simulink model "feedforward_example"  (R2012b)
settings: Solver=ode45  StartTime=0.0  StopTime=10.0  RelTol=1e-3
libraries: simulink x2

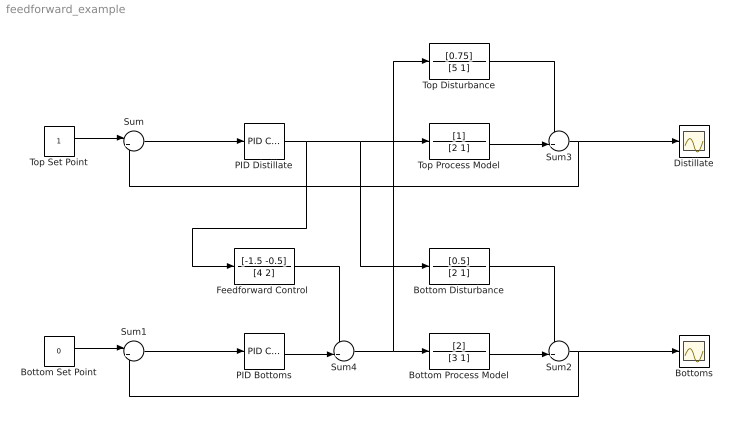
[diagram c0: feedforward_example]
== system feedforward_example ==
  Bottom Disturbance : TransferFcn  Numerator=[0.5]  Denominator=[2 1]
  Bottom Process Model : TransferFcn  Numerator=[2]  Denominator=[3 1]
  Bottom Set Point : Constant  Value=0
  Bottoms : Scope
  Distillate : Scope
  "Feedforward Control " : TransferFcn  Numerator=[-1.5 -0.5]  Denominator=[4 2]
  PID Bottoms : simulink/Continuous/PID Controller  Controller=PID  TimeDomain=Continuous-time  SampleTime=1  IntegratorMethod=Forward Euler  FilterMethod=Forward Euler  Form=Parallel  P=1  I=1  D=0  N=100  InitialConditionSource=internal  InitialConditionForIntegrator=0  InitialConditionForFilter=0  ExternalReset=none  LimitOutput=off  UpperSaturationLimit=inf  LowerSaturationLimit=-inf  LinearizeAsGain=on  AntiWindupMode=none  Kb=1  TrackingMode=off  Kt=1  PParamMin=[]  PParamMax=[]  IParamMin=[]  IParamMax=[]  DParamMin=[]  DParamMax=[]  NParamMin=[]  NParamMax=[]  KbParamMin=[]  KbParamMax=[]  KtParamMin=[]  KtParamMax=[]  POutMin=[]  POutMax=[]  IOutMin=[]  IOutMax=[]  DOutMin=[]  DOutMax=[]  NOutMin=[]  NOutMax=[]  KbOutMin=[]  KbOutMax=[]  KtOutMin=[]  KtOutMax=[]  IntegratorOutMin=[]  IntegratorOutMax=[]  FilterOutMin=[]  FilterOutMax=[]  SumOutMin=[]  SumOutMax=[]  SumI1OutMin=[]  SumI1OutMax=[]  SumI2OutMin=[]  SumI2OutMax=[]  SumI3OutMin=[]  SumI3OutMax=[]  SumDOutMin=[]  SumDOutMax=[]  SaturationOutMin=[]  SaturationOutMax=[]  IntegratorContinuousStateAttributes=''  IntegratorStateMustResolveToSignalObject=off  IntegratorRTWStateStorageClass=Auto  FilterContinuousStateAttributes=''  FilterStateMustResolveToSignalObject=off  FilterRTWStateStorageClass=Auto
  PID Distillate : simulink/Continuous/PID Controller  Controller=PID  TimeDomain=Continuous-time  SampleTime=1  IntegratorMethod=Forward Euler  FilterMethod=Forward Euler  Form=Parallel  P=1  I=1  D=0  N=100  InitialConditionSource=internal  InitialConditionForIntegrator=0  InitialConditionForFilter=0  ExternalReset=none  LimitOutput=off  UpperSaturationLimit=inf  LowerSaturationLimit=-inf  LinearizeAsGain=on  AntiWindupMode=none  Kb=1  TrackingMode=off  Kt=1  PParamMin=[]  PParamMax=[]  IParamMin=[]  IParamMax=[]  DParamMin=[]  DParamMax=[]  NParamMin=[]  NParamMax=[]  KbParamMin=[]  KbParamMax=[]  KtParamMin=[]  KtParamMax=[]  POutMin=[]  POutMax=[]  IOutMin=[]  IOutMax=[]  DOutMin=[]  DOutMax=[]  NOutMin=[]  NOutMax=[]  KbOutMin=[]  KbOutMax=[]  KtOutMin=[]  KtOutMax=[]  IntegratorOutMin=[]  IntegratorOutMax=[]  FilterOutMin=[]  FilterOutMax=[]  SumOutMin=[]  SumOutMax=[]  SumI1OutMin=[]  SumI1OutMax=[]  SumI2OutMin=[]  SumI2OutMax=[]  SumI3OutMin=[]  SumI3OutMax=[]  SumDOutMin=[]  SumDOutMax=[]  SaturationOutMin=[]  SaturationOutMax=[]  IntegratorContinuousStateAttributes=''  IntegratorStateMustResolveToSignalObject=off  IntegratorRTWStateStorageClass=Auto  FilterContinuousStateAttributes=''  FilterStateMustResolveToSignalObject=off  FilterRTWStateStorageClass=Auto
  Sum : Sum  Inputs=|+-
  Sum1 : Sum  Inputs=|+-
  Sum2 : Sum  Inputs=++|
  Sum3 : Sum  Inputs=++|
  Sum4 : Sum  Inputs=++|
  Top Disturbance : TransferFcn  Numerator=[0.75]  Denominator=[5 1]
  Top Process Model : TransferFcn  Denominator=[2 1]
  Top Set Point : Constant
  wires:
  PID Distillate/1 -> "Feedforward Control "/1, Bottom Disturbance/1, Top Process Model/1
  Sum/1 -> PID Distillate/1
  Sum1/1 -> PID Bottoms/1
  Bottom Disturbance/1 -> Sum2/1
  Top Disturbance/1 -> Sum3/1
  Top Process Model/1 -> Sum3/2
  Sum3/1 -> Distillate/1, Sum/2
  Top Set Point/1 -> Sum/1
  Bottom Set Point/1 -> Sum1/1
  Bottom Process Model/1 -> Sum2/2
  Sum2/1 -> Bottoms/1, Sum1/2
  "Feedforward Control "/1 -> Sum4/1
  PID Bottoms/1 -> Sum4/2
  Sum4/1 -> Top Disturbance/1, Bottom Process Model/1
